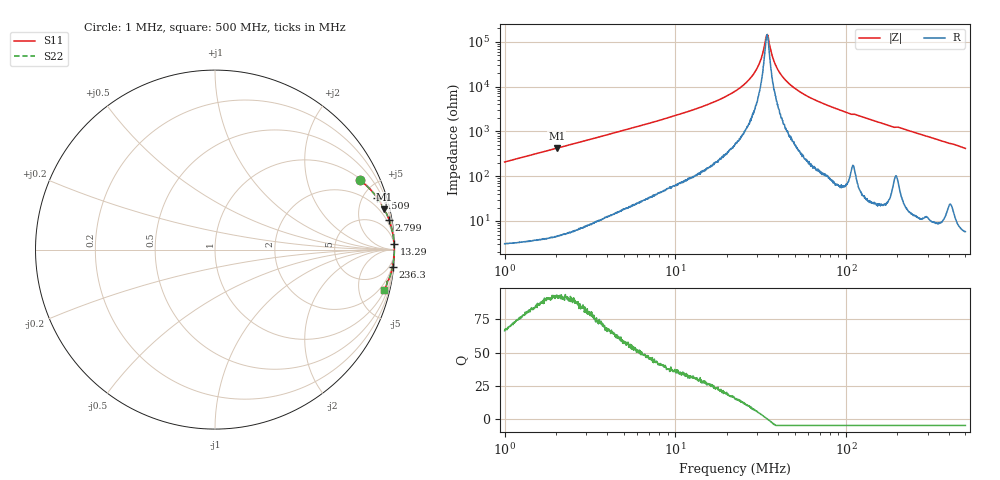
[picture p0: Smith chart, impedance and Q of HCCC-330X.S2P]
!s-Parameter Generated by FASTRON Sdn. Bhd.
!FASTRON P/N : HCCC-330X
!Keysight Technologies,E4991B,MY54100416,A.01.15
!Date: Mon Apr 06 13:09:57 2026
!Version  : Rev00 Mon Apr 06 13:09:57 2026
!Data & Calibration Information:
!PortZ  Port1:50+j0  Port2:50+j0
!When reading, reference impedance value at option line is always used.
! Remarks : This data is being provided solely for informational purposes.
!Freq	S11	S21	S12	S22
# Hz S dB R 50
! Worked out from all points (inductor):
!   1601 points, 1 MHz to 500 MHz, reference 50 ohm
!   read as one part in series: L = 33 uH near 1.032 MHz
!   highest Q = 92.8 at 2.02 MHz (marker M1), where L = 33.1 uH
!   self-resonance near 34.41 MHz
!   S11 on the Smith chart (normalised r, x): 1 MHz: 1.06, +4.15; 1.509 MHz: 1.07, +6.27; 2.799 MHz: 1, +12; 13.29 MHz: 3, +64; 236.3 MHz: 1, -20; 500 MHz: 1.12, -8.35
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1000000  -0.96 25.6  -7.30 -63.6  -7.30 -63.6  -0.96 25.6
1509408  -0.45 17.6  -10.38 -71.7  -10.38 -71.7  -0.45 17.6
2019859  -0.26 13.3  -12.74 -76.0  -12.74 -76.0  -0.26 13.3
2799090  -0.14 9.7  -15.48 -79.6  -15.48 -79.6  -0.14 9.7
2820919  -0.14 9.6  -15.55 -79.7  -15.55 -79.7  -0.14 9.6
7957584  -0.03 3.3  -24.81 -85.3  -24.81 -85.3  -0.03 3.3
1.328759e7  -0.01 1.8  -30.14 -86.3  -30.14 -86.3  -0.01 1.8
2.236068e7  -0.01 0.7  -37.91 -85.5  -37.91 -85.5  -0.01 0.7
2.601791e7  -0.01 0.5  -41.80 -84.2  -41.80 -84.2  -0.01 0.5
2.934708e7  -0.01 0.3  -46.62 -81.1  -46.62 -81.1  -0.01 0.3
3.147229e7  -0.01 0.1  -51.45 -74.5  -51.45 -74.5  -0.01 0.1
3.37514e7  -0.01 0.0  -60.75 -40.6  -60.75 -40.6  -0.01 0.0
3.441328e7  -0.01 0.0  -63.01 -5.2  -63.01 -5.2  -0.01 0.0
3.522469e7  -0.01 -0.0  -60.82 43.7  -60.82 43.7  -0.01 -0.0
3.821828e7  -0.01 -0.2  -50.44 76.6  -50.44 76.6  -0.01 -0.2
4.195229e7  -0.01 -0.3  -44.95 83.1  -44.95 83.1  -0.01 -0.3
4.957817e7  -0.01 -0.6  -39.45 85.9  -39.45 85.9  -0.01 -0.6
6.307767e7  -0.01 -1.1  -34.65 87.1  -34.65 87.1  -0.01 -1.1
1.04107e8  -0.02 -2.3  -28.01 85.8  -28.01 85.8  -0.02 -2.3
1.77937e8  -0.04 -4.2  -22.63 84.5  -22.63 84.5  -0.04 -4.2
2.36269e8  -0.05 -5.6  -20.23 83.5  -20.23 83.5  -0.05 -5.6
5e8  -0.27 -13.4  -12.68 75.8  -12.68 75.8  -0.27 -13.4
